(* Logix 5000 AddOnInstructionDefinition export B256_NEG; software revision 30.00 *)

ADD_ON_INSTRUCTION B256_NEG   (* revision 1.0 20170916, vendor Kenneth A. Fischer *)
// c2 = -c1 (mod p)
// Revision note:
// Rev1.0: 20170916 - Initial Release
VAR_OUTPUT
   FAIL : BOOL; {access Read Only}   // Indicates negative overflow which should not happen
END_VAR
VAR_IN_OUT
   Inp_C1 : DINT[22]; {required}
   Out_C2 : DINT[22]; {required}
END_VAR
VAR
   s : DINT;
   b : DINT;
   i : DINT;
END_VAR

ROUTINE Logic   (* ladder *)
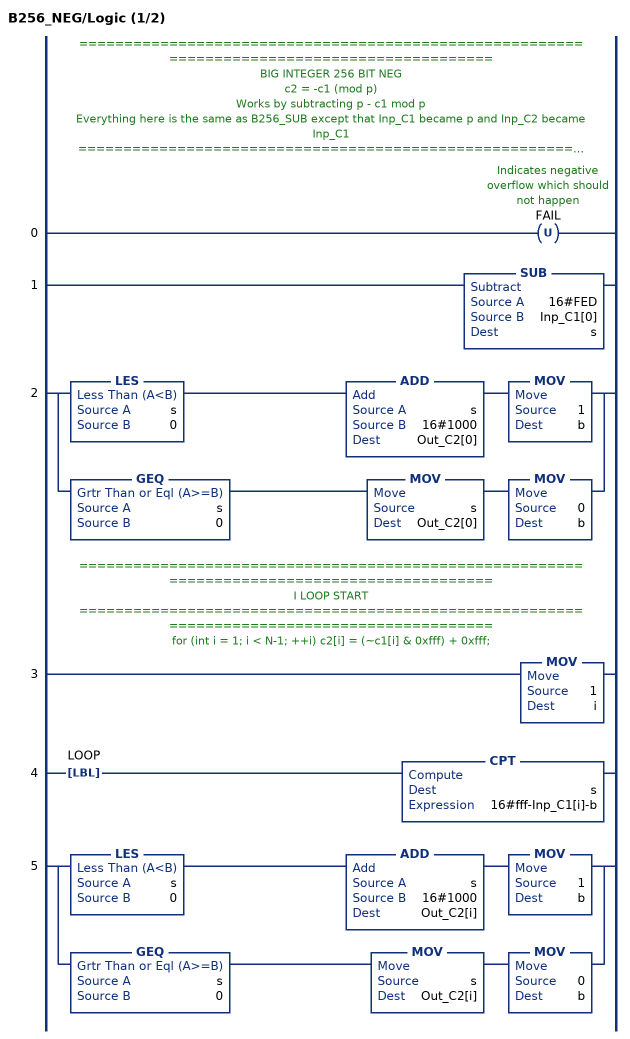
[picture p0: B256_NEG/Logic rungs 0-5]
   // ============================================================================================
   // BIG INTEGER 256 BIT NEG
   // c2 = -c1 (mod p)
   // Works by subtracting p - c1 mod p
   // Everything here is the same as B256_SUB except that Inp_C1 became p and Inp_C2 became Inp_C1
   // ============================================================================================
   0: OTU(FAIL);
   1: SUB(16#FED,Inp_C1[0],s);
   2: [LES(s,0) ADD(s,16#1000,Out_C2[0]) MOV(1,b) ,GEQ(s,0) MOV(s,Out_C2[0]) MOV(0,b) ];
   // ============================================================================================
   // I LOOP START
   // ============================================================================================
   // for (int i = 1; i < N-1; ++i) c2[i] = (~c1[i] & 0xfff) + 0xfff;
   3: MOV(1,i);
   4: LBL(LOOP)CPT(s,16#fff-Inp_C1[i]-b);
   5: [LES(s,0) ADD(s,16#1000,Out_C2[i]) MOV(1,b) ,GEQ(s,0) MOV(s,Out_C2[i]) MOV(0,b) ];
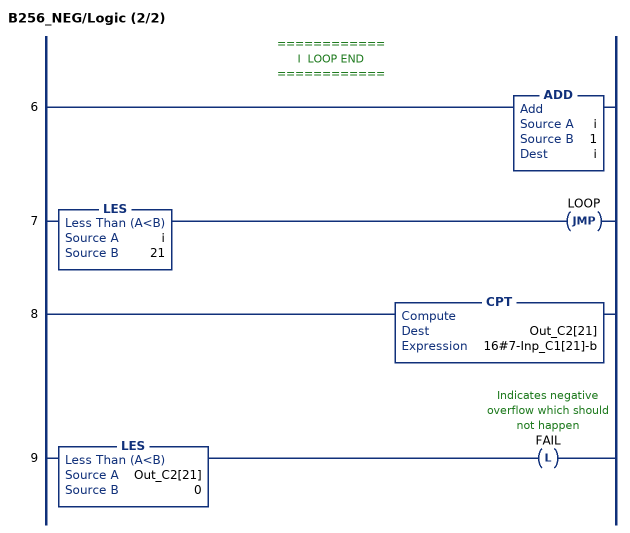
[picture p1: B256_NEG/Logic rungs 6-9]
   // ============
   // I  LOOP END
   // ============
   6: ADD(i,1,i);
   7: LES(i,21)JMP(LOOP);
   8: CPT(Out_C2[21],16#7-Inp_C1[21]-b);
   9: LES(Out_C2[21],0)OTL(FAIL);
END_ROUTINE
END_ADD_ON_INSTRUCTION
